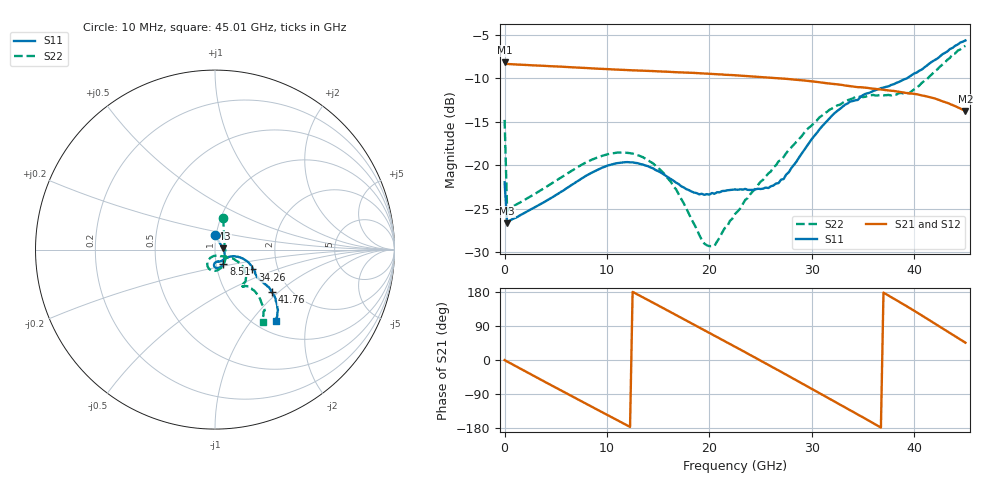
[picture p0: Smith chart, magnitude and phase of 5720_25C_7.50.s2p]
! Device:  ADRF5720
! Description: 0.5dB LSB GaAs MMIC 6-bit Digital Attenuator
! Frequency:  0.000009 -  40 GHz
! Ports:
!	RF1	= Port 1
!	RF2	= Port 2
! Vdd:  3.3 Volt
! Vss:  -3.3 Volt
! Control:  0/3.3 Volt
! State:  7.50 dB attenuation
! Data:  The device was measured using G-S-G Probes on a matrix board.
!  Data was collected using an calibrated 4 port network analyzer.
!  The reference plane for this measurement is at the launchers.
! Note:  Analog Devices supplies this data as a sample of measured data
!  for this product.  Your particular data for this product may vary.
!  Data was taken at 25 degrees C.
!  Analog Devices reserves the right to change this data at anytime.
# GHZ S DB R 45.0
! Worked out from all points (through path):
!   181 points, 10 MHz to 45.01 GHz, reference 45 ohm
!   highest |S21| = -8.16 dB at 10 MHz (marker M1); lowest = -13.7 dB at 45.01 GHz (marker M2)
!   group delay of S21, straight-line fit = 41.1 ps
!   lowest |S11| = -26.7 dB at 260 MHz (marker M3), VSWR 1.10, Z = 49.3 + j0.63 ohm
!   |S11| at or under -10 dB: start of sweep to 39.3 GHz
!   |S22| runs from -29.3 to -6.3 dB; largest |S21 - S12| = 0.00048
!   S11 on the Smith chart (normalised r, x): 10 MHz: 0.99, +0.16; 8.51 GHz: 1.08, -0.17; 34.26 GHz: 1.48, -0.35; 41.76 GHz: 1.62, -0.90; 45.01 GHz: 1.23, -1.34
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0.01  -21.95 90.5  -8.16 -0.4  -8.16 -0.4  -14.78 75.5
0.26  -26.67 7.9  -8.35 -4.0  -8.35 -4.0  -25.27 5.7
2.01  -25.43 -13.4  -8.46 -29.7  -8.46 -29.7  -23.95 -17.5
4.26  -23.96 -32.4  -8.59 -62.2  -8.59 -62.2  -22.34 -39.8
6.01  -22.67 -43.8  -8.69 -87.4  -8.69 -87.4  -21.03 -53.8
7.76  -21.35 -54.5  -8.80 -112.4  -8.80 -112.4  -19.79 -66.7
8.51  -20.85 -59.1  -8.85 -123.1  -8.85 -123.1  -19.36 -72.2
11.76  -19.64 -79.0  -9.04 -169.5  -9.04 -169.5  -18.54 -95.3
15.26  -20.82 -93.1  -9.21 140.3  -9.21 140.3  -20.57 -117.5
17.51  -22.54 -90.9  -9.33 107.9  -9.33 107.9  -24.37 -121.2
19.76  -23.31 -77.7  -9.46 75.2  -9.47 75.2  -29.19 -91.7
20.51  -23.27 -73.7  -9.52 64.3  -9.52 64.3  -29.26 -71.3
22.76  -22.81 -64.2  -9.67 31.4  -9.67 31.5  -25.30 -42.2
24.76  -22.69 -52.8  -9.82 2.1  -9.82 2.1  -22.25 -33.7
26.76  -22.04 -34.5  -9.99 -27.5  -9.99 -27.5  -19.54 -27.7
30.26  -16.62 -17.1  -10.38 -79.9  -10.39 -79.8  -15.08 -30.9
32.26  -13.98 -21.0  -10.66 -109.8  -10.67 -109.7  -13.31 -38.2
34.26  -12.53 -27.9  -10.99 -139.9  -11.00 -139.8  -12.15 -46.7
37.76  -10.76 -33.7  -11.43 166.2  -11.43 166.2  -11.97 -53.1
39.51  -9.83 -34.2  -11.74 138.2  -11.74 138.2  -11.72 -51.4
41.76  -8.08 -36.6  -12.23 100.6  -12.23 100.6  -9.52 -46.5
45.01  -5.65 -49.4  -13.74 45.8  -13.74 45.9  -6.27 -56.3
